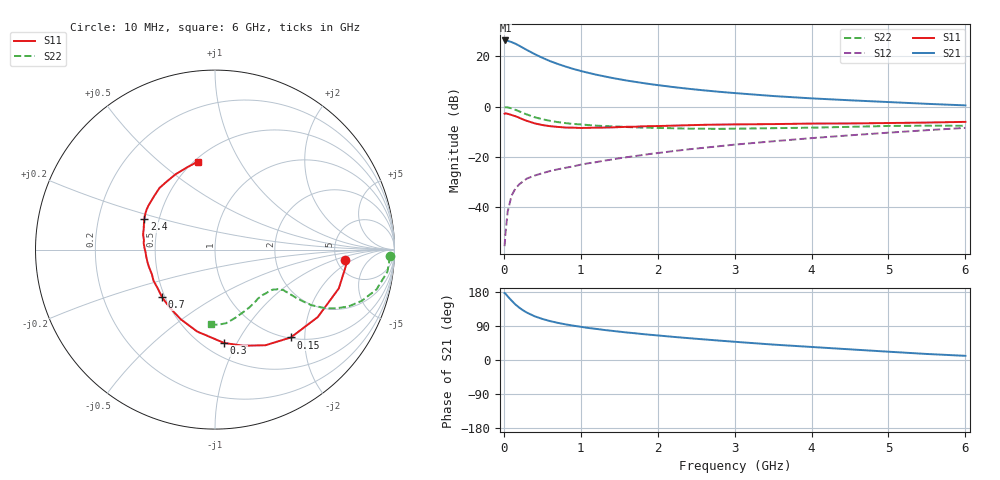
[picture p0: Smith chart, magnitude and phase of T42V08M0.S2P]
! Infineon Technologies  Discrete & RF Semiconductors
! BFR182T
! Si NPN RF Bipolar Junction Transistor in SC75
! VCE = 2 V  IC = 8 mA
! Common Emitter S-Parameters:  October  1999
# GHz  S  MA  R  50
!  f  S11  S21  S12  S22
! GHz  MAG  ANG  MAG  ANG  MAG  ANG  MAG  ANG
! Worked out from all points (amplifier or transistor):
!   36 points, 10 MHz to 6 GHz, reference 50 ohm
!   highest |S21| = 26.3 dB at 20 MHz (marker M1)
!   |S21| within 3 dB of that: start of sweep to 253.4 MHz
!   unconditionally stable (mu >= 1): 1.08 GHz to 3.846 GHz
!   at 250 MHz: K = 0.40, MSG = 26.5 dB, |S12| = -29.6 dB
!   at 1.4 GHz: K = 1.07, MAG = 14.6 dB, |S12| = -21.0 dB
!   at 6 GHz: K = 0.84, MSG = 4.5 dB, |S12| = -8.4 dB
!   lowest NFmin = 1.40 dB at 450 MHz
!   S11 on the Smith chart (normalised r, x): 10 MHz: 5.89, -1.44; 150 MHz: 1.02, -1.71; 300 MHz: 0.62, -0.89; 700 MHz: 0.48, -0.30; 2.4 GHz: 0.41, +0.17; 6 GHz: 0.52, +0.68
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0.01  0.7244 -4.6  20.54 176.7  0.0017 73.9  0.9768 -2.2
0.02  0.7384 -5.7  20.66 175.3  0.0029 95.0  0.9748 -2.9
0.05  0.7229 -17.4  20.28 167.9  0.0083 85.6  0.9685 -7.3
0.1  0.6849 -33.3  19.18 156.9  0.0171 76.7  0.9266 -13.9
0.15  0.6467 -49.2  17.79 146.6  0.0236 69.3  0.8664 -19.2
0.2  0.6025 -62.2  16.25 138.2  0.0287 65.9  0.8079 -23.1
0.25  0.5582 -73.6  14.72 131.1  0.033 60.7  0.7489 -25.9
0.3  0.5227 -84.4  13.34 125.0  0.0374 59.5  0.7003 -27.9
0.4  0.4671 -102.3  11.09 115.4  0.0429 56.8  0.6178 -30.0
0.5  0.4325 -116.2  9.364 108.4  0.0477 55.7  0.5641 -30.5
0.6  0.4101 -127.8  8.046 102.7  0.0528 56.1  0.5243 -30.7
0.7  0.3971 -137.9  7.064 98.1  0.0571 56.0  0.4942 -30.7
0.9  0.3838 -153.2  5.633 90.7  0.0652 58.8  0.4543 -30.7
1.1  0.3806 -165.2  4.694 84.5  0.0753 60.6  0.4316 -31.2
1.3  0.3852 -174.4  4.022 79.4  0.0847 61.5  0.413 -32.2
1.6  0.3989 174.9  3.302 72.6  0.0994 63.1  0.3944 -34.3
2.2  0.4203 160.4  2.456 61.1  0.1311 64.6  0.3733 -40.9
2.4  0.4286 156.7  2.268 57.7  0.1423 64.8  0.3668 -43.5
3.5  0.4512 138.8  1.629 40.7  0.2056 62.9  0.3743 -58.8
4.5  0.4649 125.3  1.34 28.1  0.2702 58.9  0.3978 -74.0
5.5  0.4839 108.8  1.14 15.9  0.3418 53.3  0.4189 -87.4
6  0.4996 100.9  1.061 11.0  0.3796 49.7  0.4177 -92.9
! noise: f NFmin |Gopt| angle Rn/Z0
0.45  1.4  0.26  41  0.29
0.9  1.5  0.25  83  0.23
1.8  2  0.21  162  0.2
